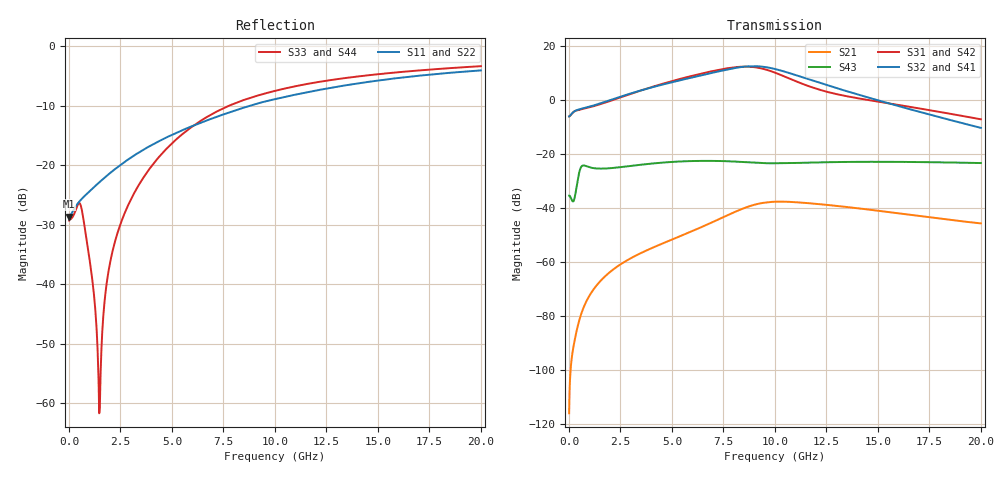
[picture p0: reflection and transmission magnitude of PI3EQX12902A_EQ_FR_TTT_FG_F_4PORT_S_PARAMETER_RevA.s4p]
! NPort=4 DATA=2000 NOISE=0 GROUPDELAY=0 COMPLEX_DATAFORMAT=POLAR
! NumOfBlock=1 NumOfParam=0
! .MODEL Smodel S TSTONEFILE=PI3EQX12902A_EQ_FR_TTT_FG_F_4PORT_S_PARAMETER_RevA.s4p TYPE=S
!  -- The above .MODEL line can be used for the S element in the netlist.
! The s parameter is extracted from the linear redriver, it is not bi-directional; only s(4,1)s(4,2) and s(3,1)s(3,2)
! should be the insertion loss
!Port definition:
!Port1 = input+
!Port2 = input-
!Port3 = output+
!Port4 = output-
# Hz S MA R  50
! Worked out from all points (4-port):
!   2000 points, 10 MHz to 20 GHz, reference 50 ohm
!   strongest paths, dB at 10 MHz, 5.01 GHz, 10.01 GHz, 15.01 GHz, 20 GHz:
!     S32: -6.0, 6.6, 11.5, -0.1, -10.3
!     S41: -6.0, 6.6, 11.4, -0.1, -10.3
!     S31: -6.0, 7.0, 10.2, -0.6, -7.1
!     S42: -6.0, 7.0, 10.0, -0.8, -7.2
!     S43: -35.3, -22.9, -23.4, -22.8, -23.3
!     S21: -116.0, -51.6, -37.6, -41.0, -45.7
!   lowest |S11| = -28.6 dB at 10 MHz (marker M1), VSWR 1.08, Z = 46.4 - j0.0607 ohm
!   |S11| at or under -10 dB: start of sweep to 8.792 GHz
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1e7  0.03704 -179.0  1.589e-06 51.9  0 0.0  0 0.0
     1.589e-06 51.9  0.03704 -179.0  0 0.0  0 0.0
     0.4992 1.0  0.4992 -179.0  0.03429 6.0  0.01709 -177.1
     0.4992 -179.0  0.4992 1.0  0.01709 -177.1  0.03429 6.0
5.93e9  0.2112 -112.0  0.00368 97.1  1.573e-06 -21.7  9.829e-07 88.3
        0.003677 97.1  0.2112 -112.0  9.851e-07 88.4  1.566e-06 -21.4
        2.785 -48.3  2.598 111.5  0.2078 -45.7  0.07394 145.4
        2.589 111.5  2.749 -48.8  0.07433 145.5  0.2072 -45.8
7.83e9  0.2796 -111.7  0.007793 78.9  6.433e-06 -78.6  4.091e-06 44.4
        0.007779 78.8  0.2796 -111.7  4.101e-06 44.4  6.403e-06 -78.2
        3.961 -101.7  3.784 57.7  0.319 -64.6  0.07299 125.3
        3.761 57.7  3.897 -102.1  0.07347 125.2  0.3184 -64.5
9.2e9  0.3316 -113.3  0.01208 48.1  1.194e-05 -126.5  9.577e-06 -4.7
       0.01205 48.1  0.3316 -113.3  9.572e-06 -4.8  1.19e-05 -125.9
       3.962 -153.4  4.221 4.4  0.3862 -75.8  0.06838 114.8
       4.183 4.4  3.89 -153.8  0.06879 114.6  0.3858 -75.6
1.065e10  0.3805 -115.7  0.01313 11.8  1.524e-05 -165.8  1.476e-05 -61.5
          0.01309 12.0  0.3806 -115.7  1.47e-05 -61.5  1.526e-05 -165.0
          2.56 160.2  3.211 -50.6  0.4477 -85.3  0.06773 107.7
          3.175 -50.3  2.503 159.9  0.06798 107.4  0.4477 -85.2
1.305e10  0.4575 -119.5  0.01095 -26.9  2.266e-05 154.2  1.869e-05 -131.7
          0.01094 -26.5  0.4576 -119.5  1.855e-05 -131.5  2.286e-05 154.8
          1.277 125.3  1.643 -112.7  0.5294 -97.8  0.07132 92.0
          1.628 -112.0  1.245 125.6  0.07129 91.8  0.5298 -97.7
2e10  0.6262 -131.6  0.005159 -75.0  4.123e-05 50.7  1.797e-05 98.8
      0.005216 -75.0  0.6261 -131.6  1.777e-05 99.7  4.17e-05 50.9
      0.4414 38.8  0.3058 132.0  0.6794 -119.6  0.06844 46.2
      0.3069 132.9  0.4364 39.6  0.06834 46.1  0.6797 -119.6
